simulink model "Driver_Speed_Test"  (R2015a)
settings: Solver=ode45  StartTime=0.0  StopTime=10.0  RelTol=1e-3
undefined symbols (not defined in the file or in its folder): Vsupply
libraries: arduinolib x4, RASPlib x3, simulink x2, MinSegLibrary_MinSegMega x2

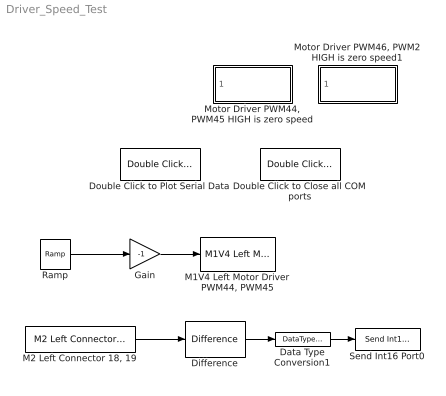
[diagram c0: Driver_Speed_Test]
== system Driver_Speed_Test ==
  Data Type Conversion1 : DataTypeConversion  OutDataTypeStr=int16
  Difference : simulink/Discrete/Difference  ICPrevInput=0.0  InputProcessing=Inherited  OutMin=[]  OutMax=[]  OutDataType=fixdt(1, 16)  OutScaling=2^-10  DoSatur=off
  Double Click to Close all COM ports : RASPlib/Double Click to Close all COM ports
  Double Click to Plot Serial Data : RASPlib/Double Click to Plot Serial Data  COMport=127  BaudRate=9600  NumSamples=500  DataType=int16
  Gain : Gain  Gain=-1
  "M1V4 Left Motor Driver PWM44, PWM45" : MinSegLibrary_MinSegMega/M1V4 Left Motor Driver PWM44, PWM45  Vsupply=3.9  PWMoffset=0
  "M2 Left Connector 18, 19" : MinSegLibrary_MinSegMega/M2 Left Connector 18, 19  Encoder=1  PinA=19  PinB=18  PWMFSelect=1  PWMTimer=3  SampleTime=-1
  "Motor Driver PWM44, PWM45 HIGH is zero speed" : Subsystem  Commented=on
  "Motor Driver PWM46, PWM2 HIGH is zero speed1" : Subsystem  Commented=on
  Ramp : simulink/Sources/Ramp  slope=.05  start=0  X0=0
  Send Int16 Port0 : RASPlib/Send Int16 Port0
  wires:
  Ramp/1 -> Gain/1
  Difference/1 -> Data Type Conversion1/1
  "M2 Left Connector 18, 19"/1 -> Difference/1
  Data Type Conversion1/1 -> Send Int16 Port0/1
  Gain/1 -> "M1V4 Left Motor Driver PWM44, PWM45"/1

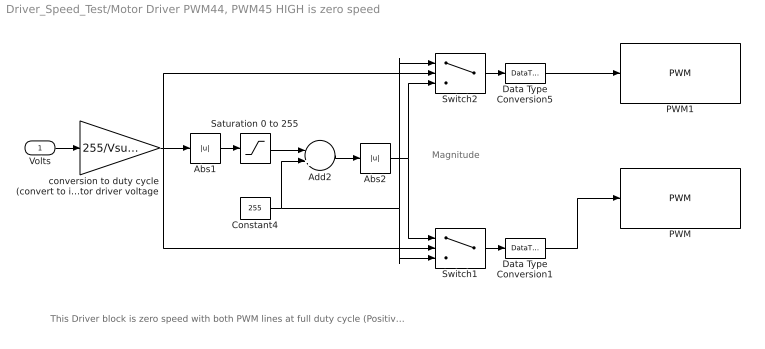
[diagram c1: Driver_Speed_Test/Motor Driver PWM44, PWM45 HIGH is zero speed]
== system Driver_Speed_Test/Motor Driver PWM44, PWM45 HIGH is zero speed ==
  note: This Driver block is zero speed with both PWM lines at full duty cycle (Positive voltage on both motor terminals). This method produces a linear motor response for DRV8833 driver in both directions and eliminates the typical dead zone when the motor starts. The driver may draw more current in this configuration (has not been verified) The SN754410 driver this has no effect, so the driver could alternatively be modified so that zero speed is zero voltage to both PWM lines.
  note: Magnitude
  Volts : Inport
  Abs1 : Abs
  Abs2 : Abs
  Add2 : Sum  Inputs=-+
  Constant4 : Constant  Value=255
  Data Type Conversion1 : DataTypeConversion  OutDataTypeStr=uint8
  Data Type Conversion5 : DataTypeConversion  OutDataTypeStr=uint8
  PWM : arduinolib/PWM  pinNumber=45  blockPlatform=arduino
  PWM1 : arduinolib/PWM  pinNumber=44  blockPlatform=arduino
  Saturation 0 to 255 : Saturate  UpperLimit=255  LowerLimit=0
  Switch1 : Switch
  Switch2 : Switch
  conversion to duty cycle (convert to int) denominator is motor driver voltage : Gain  Gain=255/Vsupply  OutDataTypeStr=int16
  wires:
  Volts/1 -> conversion to duty cycle (convert to int) denominator is motor driver voltage/1
  conversion to duty cycle (convert to int) denominator is motor driver voltage/1 -> Switch2/2, Abs1/1, Switch1/2
  Saturation 0 to 255/1 -> Add2/1
  Abs1/1 -> Saturation 0 to 255/1
  Constant4/1 -> Switch1/3, Switch2/1, Add2/2
  Add2/1 -> Abs2/1
  Abs2/1 -> Switch2/3, Switch1/1
  Switch2/1 -> Data Type Conversion5/1
  Switch1/1 -> Data Type Conversion1/1
  Data Type Conversion5/1 -> PWM1/1
  Data Type Conversion1/1 -> PWM/1

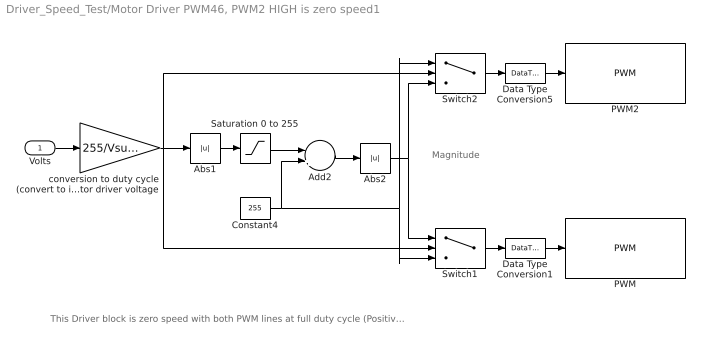
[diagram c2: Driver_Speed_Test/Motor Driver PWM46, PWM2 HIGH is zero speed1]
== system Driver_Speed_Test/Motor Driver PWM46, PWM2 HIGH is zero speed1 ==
  note: This Driver block is zero speed with both PWM lines at full duty cycle (Positive voltage on both motor terminals). This method produces a linear motor response for DRV8833 driver in both directions and eliminates the typical dead zone when the motor starts. The driver may draw more current in this configuration (has not been verified) The SN754410 driver this has no effect, so the driver could alternatively be modified so that zero speed is zero voltage to both PWM lines.
  note: Magnitude
  Volts : Inport
  Abs1 : Abs
  Abs2 : Abs
  Add2 : Sum  Inputs=-+
  Constant4 : Constant  Value=255
  Data Type Conversion1 : DataTypeConversion  OutDataTypeStr=uint8
  Data Type Conversion5 : DataTypeConversion  OutDataTypeStr=uint8
  PWM : arduinolib/PWM  pinNumber=2  blockPlatform=arduino
  PWM2 : arduinolib/PWM  pinNumber=46  blockPlatform=arduino
  Saturation 0 to 255 : Saturate  UpperLimit=255  LowerLimit=0
  Switch1 : Switch
  Switch2 : Switch
  conversion to duty cycle (convert to int) denominator is motor driver voltage : Gain  Gain=255/Vsupply  OutDataTypeStr=int16
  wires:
  Volts/1 -> conversion to duty cycle (convert to int) denominator is motor driver voltage/1
  conversion to duty cycle (convert to int) denominator is motor driver voltage/1 -> Abs1/1, Switch2/2, Switch1/2
  Saturation 0 to 255/1 -> Add2/1
  Abs1/1 -> Saturation 0 to 255/1
  Constant4/1 -> Switch1/3, Switch2/1, Add2/2
  Add2/1 -> Abs2/1
  Abs2/1 -> Switch2/3, Switch1/1
  Switch2/1 -> Data Type Conversion5/1
  Switch1/1 -> Data Type Conversion1/1
  Data Type Conversion5/1 -> PWM2/1
  Data Type Conversion1/1 -> PWM/1
